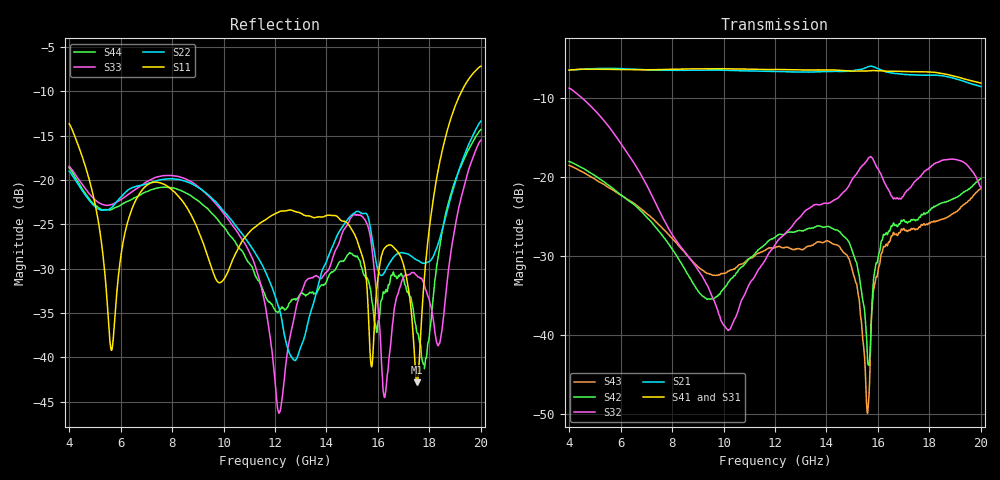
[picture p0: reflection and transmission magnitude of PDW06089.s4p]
!Keysight Technologies,N5247B,US57180241,A.12.85.04
!Date: Friday, March 23, 2018 09:51:30
!Correction: S11(Full 4 Port(1,2,3,4))
!S12(Full 4 Port(1,2,3,4))
!S13(Full 4 Port(1,2,3,4))
!S14(Full 4 Port(1,2,3,4))
!S21(Full 4 Port(1,2,3,4))
!S22(Full 4 Port(1,2,3,4))
!S23(Full 4 Port(1,2,3,4))
!S24(Full 4 Port(1,2,3,4))
!S31(Full 4 Port(1,2,3,4))
!S32(Full 4 Port(1,2,3,4))
!S33(Full 4 Port(1,2,3,4))
!S34(Full 4 Port(1,2,3,4))
!S41(Full 4 Port(1,2,3,4))
!S42(Full 4 Port(1,2,3,4))
!S43(Full 4 Port(1,2,3,4))
!S44(Full 4 Port(1,2,3,4))
!S4P File: Measurements: <S11,S12,S13,S14>,
!<S21,S22,S23,S24>,
!<S31,S32,S33,S34>,
!<S41,S42,S43,S44>:
# Hz S  dB  R 50
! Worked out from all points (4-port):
!   6401 points, 4 GHz to 20 GHz, reference 50 ohm
!   strongest paths, dB at 4 GHz, 8 GHz, 12 GHz, 16 GHz, 20 GHz:
!     S41: -6.4, -6.3, -6.3, -6.5, -8.1
!     S31: -6.5, -6.3, -6.4, -6.6, -8.0
!     S21: -6.4, -6.4, -6.6, -6.2, -8.5
!     S32: -8.7, -27.2, -28.6, -18.9, -21.3
!     S42: -18.0, -29.1, -27.6, -30.3, -20.2
!     S43: -18.5, -27.8, -28.9, -32.0, -21.4
!   lowest |S11| = -42.8 dB at 17.52 GHz (marker M1), VSWR 1.01, Z = 50 + j0.723 ohm
!   |S11| at or under -10 dB: start of sweep to 19.25 GHz
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4e9  -13.65 26.4  -6.45 -147.4  -6.54 -149.1  -6.41 -148.2
     -6.40 -147.2  -19.00 -18.6  -8.71 -116.5  -17.95 125.2
     -6.49 -149.1  -8.70 -116.6  -18.43 -21.0  -18.45 123.8
     -6.41 -148.3  -18.00 124.9  -18.49 123.7  -18.62 -20.3
5.6425e9  -39.19 44.8  -6.20 145.4  -6.25 143.5  -6.30 144.4
          -6.19 145.5  -23.11 -22.3  -14.00 -162.1  -21.24 34.4
          -6.25 143.4  -14.02 -162.2  -22.76 -30.9  -21.49 29.7
          -6.32 144.3  -21.28 34.2  -21.52 29.7  -23.32 -27.0
1.01725e10  -30.33 166.3  -6.46 -44.8  -6.34 -46.7  -6.21 -44.6
            -6.45 -45.0  -24.04 -128.2  -39.45 -128.9  -33.32 24.1
            -6.30 -47.2  -39.42 -128.9  -24.38 -125.5  -31.83 43.8
            -6.25 -44.7  -33.37 24.2  -31.91 44.2  -25.97 -145.2
1.21625e10  -23.56 60.2  -6.57 -132.8  -6.48 -135.6  -6.29 -132.9
            -6.59 -132.8  -34.47 173.9  -27.85 -85.7  -27.19 -123.9
            -6.47 -135.7  -27.83 -85.9  -46.27 -89.1  -28.71 -111.5
            -6.34 -132.8  -27.23 -123.8  -28.77 -111.3  -34.74 105.4
1.56025e10  -33.49 -26.1  -5.98 63.6  -6.60 60.2  -6.50 62.3
            -6.00 64.2  -24.03 -70.8  -17.70 -139.5  -43.52 33.7
            -6.61 61.1  -17.69 -139.2  -25.12 -95.6  -49.75 -93.2
            -6.52 63.6  -43.53 34.2  -49.82 -91.3  -31.20 -104.6
1.7525e10  -42.82 87.7  -6.95 -39.6  -6.99 -39.6  -6.64 -37.2
           -7.04 -39.2  -29.02 -108.9  -20.48 -158.0  -25.53 -41.0
           -6.87 -39.9  -20.26 -158.7  -30.80 -20.2  -26.48 -41.2
           -6.62 -36.8  -25.42 -41.2  -26.59 -40.6  -37.25 15.9
2e10  -7.15 57.7  -8.22 179.9  -8.07 -176.7  -8.08 -174.1
      -8.50 179.2  -13.36 65.9  -21.64 136.2  -20.48 150.7
      -8.00 -179.0  -21.30 134.6  -15.50 43.9  -21.37 145.7
      -8.06 -176.1  -20.18 149.5  -21.43 146.2  -14.29 49.8
